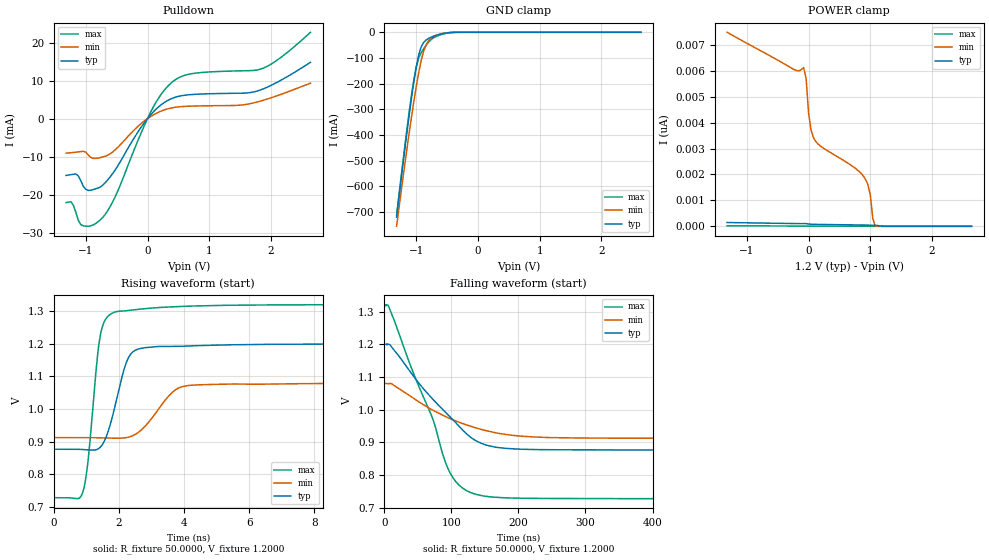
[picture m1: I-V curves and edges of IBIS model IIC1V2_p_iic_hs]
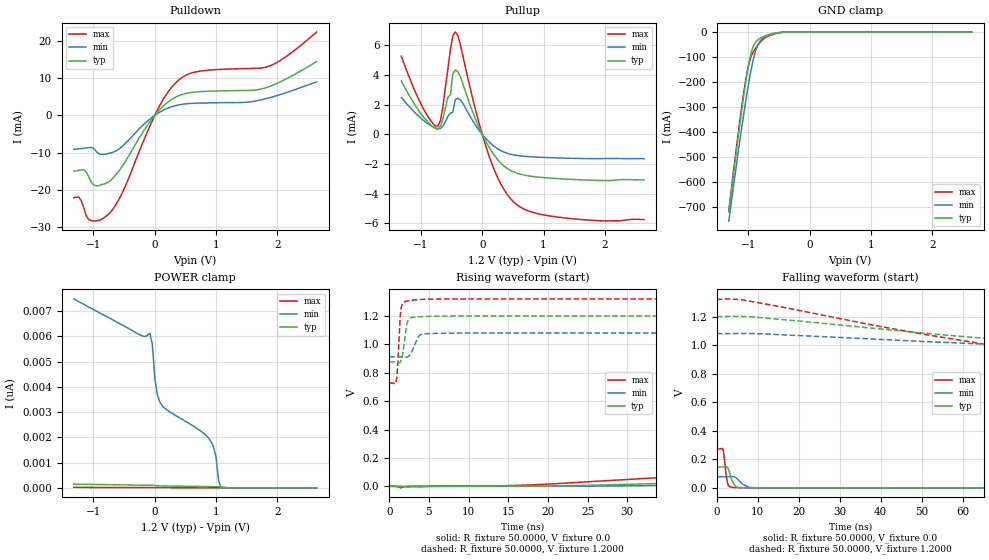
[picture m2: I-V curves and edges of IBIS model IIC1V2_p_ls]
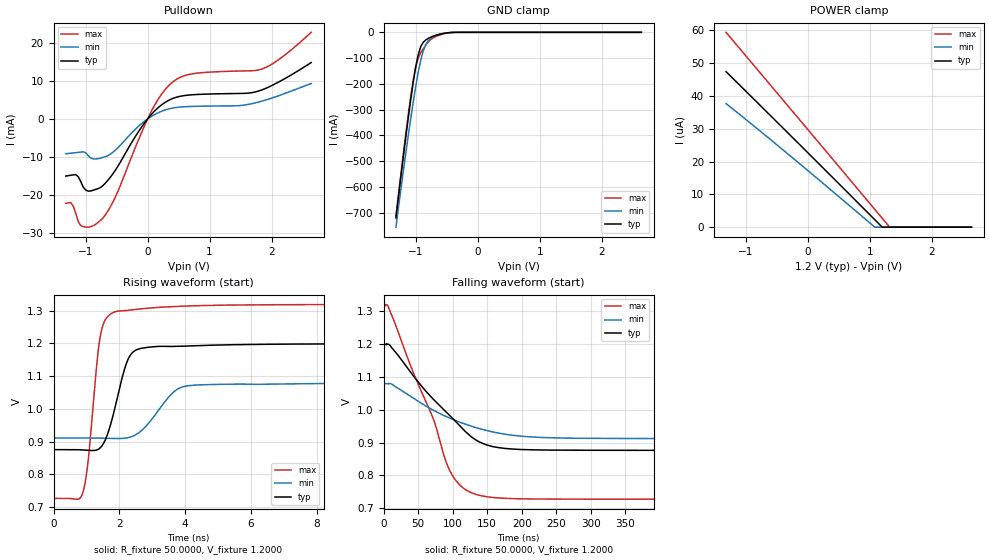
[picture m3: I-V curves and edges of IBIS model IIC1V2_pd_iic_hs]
| IBIS file qfn48_1p2v.ibs generated by Viper version: 2020.12.17
[IBIS Ver]   5.0
[Comment Char]   |_char
[File Name]   qfn48_1p2v.ibs
[File Rev]   1.3
[Date]   Thu Dec 17 17:48:23 2020
[Source]   NXP Viper 2020.12.17
[Notes]
[Disclaimer] IMPORTANT NOTICE
  This information is provided on an AS IS basis and without warranty.
  IN NO EVENT SHALL NXP BE LIABLE FOR INCIDENTAL OR CONSEQUENTIAL
  DAMAGES ARISING FROM USE OF THIS INFORMATION. THIS DISCLAIMER OF
  WARRANTY EXTENDS TO THE USER OF THE INFORMATION, AND TO THEIR CUSTOMERS
  OR USERS OF PRODUCTS  AND IS IN LIEU OF ALL WARRANTIES WHETHER EXPRESS,
  IMPLIED, OR STATUTORY, INCLUDING IMPLIED WARRANTIES OF MERCHANTABILITY
  OR FITNESS FOR PARTICULAR PURPOSE.
  NXP does not represent or warrant that the information furnished
  hereunder is free of infringement of any third party patents,
  copyrights, trade secrets, or other intellectual property rights.
  NXP does not represent or warrant that the information is free of
  defect, or that it meets any particular standard, requirements or need
  of the user of the infomation or their customers.
  NXP reserves the right to change the information in this file
  without notice.
   http://www.nxp.com
[Copyright]   (C) Copyright NXP 2004 - 2020, All Rights Reserved.
|   qfn48
[Component]   qfn48
[Manufacturer]   NXP
[Package]
| variable   typ   min   max
R_pkg   0.17546   0.085233   0.21913
L_pkg   1.979e-9   1.305e-9   2.456e-9
C_pkg   2.005e-13   1.705e-13   3.136e-13
[Pin] signal_name   model_name   R_pin   L_pin   C_pin
1   OPAMP2_INN   NC   0.19686   2.31e-9   1.975e-13
2   P0_1   gpio   0.19885   2.125e-9  1.995e-13
3   P1_0   gpio   0.18462   1.924e-9  1.916e-13
4   P0_11   gpio   0.16868   1.868e-9  1.705e-13
5   VDDIO_1   POWER   NA   NA   NA
6   VDDA   POWER   NA   NA   NA
7   VREF_OUT   NC   0.085233  1.305e-9  2.26e-13
8   VREFP   NC   0.088717  1.309e-9  2.417e-13
9   VREFN   GND   NA   NA   NA
10   P0_16   gpio   0.17435   1.987e-9  1.764e-13
11   P0_10   gpio   0.18496   2.194e-9  1.962e-13
12   P0_15   gpio   0.20527   2.456e-9  2.081e-13
13   P0_8   gpio   0.19119   2.293e-9  1.955e-13
14   OPAMP0_INN   NC   0.1741   2.073e-9  2.101e-13
15   P0_27   gpio   0.16311   1.909e-9  1.814e-13
16   OPAMP1_INN   NC   0.16129   1.801e-9  1.909e-13
17   RESETN   gpio   0.16527   1.717e-9  1.895e-13
18   VDD_CORE   POWER   NA   NA   NA
19   P0_17   gpio   0.16074   1.801e-9  1.861e-13
20   P0_7   gpio   0.1631   1.762e-9  1.925e-13
21   VDDIO_1   POWER   NA   NA   NA
22   VSS_MAIN   GND   NA   NA   NA
23   LX   NC   0.10755   1.361e-9  3.136e-13
24   VDD_MAIN_PWR   NC   NA   NA   NA
25   VBAT   NC   0.21039   2.199e-9  2.126e-13
26   P0_0   gpio   0.19752   2.015e-9  2.122e-13
27   P0_9   gpio   0.17432   1.951e-9  1.886e-13
28   P0_18   gpio   0.16396   1.852e-9  1.719e-13
29   P1_1   gpio   0.1654   1.786e-9  1.75e-13
30   P0_26   gpio   0.16144   1.856e-9  1.764e-13
31   P1_2   gpio   0.16991   1.948e-9  1.848e-13
32   P1_3   gpio   0.18887   2.054e-9  1.928e-13
33   P0_24   gpio   0.17001   1.885e-9  1.791e-13
34   P0_13   iic   0.18016   2.084e-9  1.944e-13
35   P0_14   iic   0.19867   2.298e-9  2.017e-13
36   P0_20   gpio   0.21913   2.324e-9  2.127e-13
37   P0_21   gpio   0.20869   2.216e-9  2.193e-13
38   P0_2   gpio   0.21473   2.265e-9  2.308e-13
39   P0_19   gpio   0.18997   2.14e-9   2.172e-13
40   P0_3   gpio   0.17488   1.926e-9  2.022e-13
41   VDDIO_2   POWER   NA   NA   NA
42   P0_4   gpio   0.16342   1.796e-9  1.814e-13
43   P0_6   gpio   0.16772   1.736e-9  1.992e-13
44   P0_5   gpio   0.16504   1.891e-9  1.879e-13
45   P0_29   gpio   0.16929   1.996e-9  1.98e-13
46   P1_11   gpio   0.18558   2.171e-9  1.964e-13
47   P0_30   gpio   0.20664   2.318e-9  2.205e-13
48   P2_1   gpio   0.1989   2.278e-9  1.972e-13
49   VSS   GND   NA   NA   NA
[Pin Mapping]   pulldown_ref   pullup_ref
1   NC   NC
2   VSS   VDDA
3   VSS   VDDA
4   VSS   VDDA
5   NC   VDDIO_1
6   NC   VDDA
7   NC   NC
8   NC   NC
9   VREFN   NC
10   VSS   VDDA
11   VSS   VDDA
12   VSS   VDDA
13   VSS   VDDA
14   NC   NC
15   VSS   VDDA
16   NC   NC
17   VSS   VDDIO_1
18   NC   VDD_CORE
19   VSS   VDDIO_1
20   VSS   VDDIO_1
21   NC   VDDIO_1
22   VSS_MAIN   NC
23   NC   NC
24   NC   NC
25   NC   NC
26   VSS   VDDIO_2
27   VSS   VDDIO_2
28   VSS   VDDIO_2
29   VSS   VDDIO_2
30   VSS   VDDIO_2
31   VSS   VDDIO_2
32   VSS   VDDIO_2
33   VSS   VDDIO_2
34   VSS   VDDIO_2
35   VSS   VDDIO_2
36   VSS   VDDIO_2
37   VSS   VDDIO_2
38   VSS   VDDIO_2
39   VSS   VDDIO_2
40   VSS   VDDIO_2
41   NC   VDDIO_2
42   VSS   VDDIO_2
43   VSS   VDDIO_2
44   VSS   VDDIO_2
45   VSS   VDDIO_2
46   VSS   VDDIO_2
47   VSS   VDDIO_2
48   VSS   VDDA
49   VSS   NC
|*   Model Selector   *
[Model Selector] gpio
MFIO1V2_pd_hs   EPUN=1 EPD=1 EHS=1
MFIO1V2_pd_ls   EPUN=1 EPD=1 EHS=0
MFIO1V2_pu_hs   EPUN=0 EPD=0 EHS=1
MFIO1V2_pu_ls   EPUN=0 EPD=0 EHS=0
MFIO1V2_p_hs   EPUN=1 EPD=0 EHS=1
MFIO1V2_p_ls   EPUN=1 EPD=0 EHS=0
MFIO1V2_r_hs   EPUN=0 EPD=1 EHS=1
MFIO1V2_r_ls   EPUN=0 EPD=1 EHS=0
[Model Selector] iic
IIC1V2_pd_hs   EGP=1 EPUN=1 EPD=1 EHS=1
IIC1V2_pd_ls   EGP=1 EPUN=1 EPD=1 EHS=0
IIC1V2_p_hs   EGP=1 EPUN=1 EPD=0 EHS=1
IIC1V2_p_ls   EGP=1 EPUN=1 EPD=0 EHS=0
IIC1V2_pu_hs   EGP=1 EPUN=0 EPD=0 EHS=1
IIC1V2_pu_ls   EGP=1 EPUN=0 EPD=0 EHS=0
IIC1V2_r_hs   EGP=1 EPUN=0 EPD=1 EHS=1
IIC1V2_r_ls   EGP=1 EPUN=0 EPD=1 EHS=0
IIC1V2_pd_iic_hs   EGP=0 ECS=0 EPUN=1 EPD=1
IIC1V2_p_iic_hs   EGP=0 ECS=0 EPUN=1 EPD=0
IIC1V2_pu_iic_hs   EGP=0 ECS=0 EPUN=0 EPD=0
IIC1V2_r_iic_hs   EGP=0 ECS=0 EPUN=0 EPD=1
IIC1V2_pd_iic_pu_hs   EGP=0 ECS=1 EPUN=1 EPD=1 SSEL=1
IIC1V2_p_iic_pu_hs   EGP=0 ECS=1 EPUN=1 EPD=0 SSEL=1
IIC1V2_pu_iic_pu_hs   EGP=0 ECS=1 EPUN=0 EPD=0 SSEL=1
IIC1V2_r_iic_pu_hs   EGP=0 ECS=1 EPUN=0 EPD=1 SSEL=1
| End [Component] qfn48
| Models and submodels in the file (24): IIC1V2_p_hs (I/O), IIC1V2_p_iic_hs (I/O_open_drain), IIC1V2_p_iic_pu_hs (I/O_open_drain), IIC1V2_p_ls (I/O), IIC1V2_pd_hs (I/O), IIC1V2_pd_iic_hs (I/O_open_drain), IIC1V2_pd_iic_pu_hs (I/O_open_drain), IIC1V2_pd_ls (I/O), IIC1V2_pu_hs (I/O), IIC1V2_pu_iic_hs (I/O_open_drain), IIC1V2_pu_iic_pu_hs (I/O_open_drain), IIC1V2_pu_ls (I/O), IIC1V2_r_hs (I/O), IIC1V2_r_iic_hs (I/O_open_drain), IIC1V2_r_iic_pu_hs (I/O_open_drain), IIC1V2_r_ls (I/O), MFIO1V2_p_hs (I/O), MFIO1V2_p_ls (I/O), MFIO1V2_pd_hs (I/O), MFIO1V2_pd_ls (I/O), MFIO1V2_pu_hs (I/O), MFIO1V2_pu_ls (I/O), MFIO1V2_r_hs (I/O), MFIO1V2_r_ls (I/O)
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[Model] IIC1V2_p_iic_hs
|   Model IIC1V2_p_iic_hs
| This model was characterised for following simulation conditions:
| External (pad) voltage:
|   - Typ: 1.2V,   - Min: 1.08V,   - Max: 1.32V
| Library cells for typ/min/max conditions are connected as defined below:
|  IO - External Pad
|  A - Core Input
|  EN - Output Buffer Enable
|  BOOST - vdde
|  ECS - gnd
|  EGP - gnd
|  ENZI - vdd
|  EPD - gnd
|  EPUN - vdd
|  ZI - NC
|  ZIF - NC
|  gnd - gnd
|  gnde - gnde
|  vdd - vdd
|  vdde - vdde
| All other pins connected to ground
Model_type I/O_open_drain
Polarity   Non-Inverting
Enable   Active-Low
Vinl =   0.5400V
Vinh =   1.2600V
Vmeas =  0.9000V
Cref =   0.0F
Rref =   1.0000k
Vref =   1.2000V
C_comp   3.6477pF   3.5140pF   3.7674pF
|C_comp_pullup   0.9543pF   0.9094pF   0.9729pF
|C_comp_pulldown   2.3399pF   2.4911pF   2.1962pF
[Model Spec]
| variable   typ   min   max
Vinh   0.3600V   0.3240V   0.3960V
Vinl   0.8400V   0.7560V   0.9240V
Vmeas   0.6000V   0.5400V   0.6600V
Vref   1.2000V   1.0800V   1.3200V
Cref   0.0F   0.0F   0.0F
Rref   1.0000k   1.0000k   1.0000k
[Temperature Range]   25.0000   0.1250k   -40.0000
[Voltage Range]   1.2000V   1.0800V   1.3200V
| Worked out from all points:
|   slope of the pulldown table from 0 to 0.18 V, typ, clamps not added: 58.3 ohm
|   GND clamp passes 1 mA (typ) near -0.45 V on its own axis
|   rising waveform, R_fixture 50.0000, V_fixture 1.2000: 20-80 % time 502ps typ, 802ps min, 333ps max; typ from 0.877 V to 1.2 V
|   falling waveform, R_fixture 50.0000, V_fixture 1.2000: 20-80 % time 83.3ns typ, 98.9ns min, 62.7ns max; typ from 1.2 V to 0.877 V
[Pulldown]
|Voltage   I(typ)   I(min)   I(max)
-1.32V    -14.96mA   -9.099mA   -22.09mA
-1.24V    -14.75mA   -8.982mA   -21.89mA
-1.16V    -14.56mA   -8.83mA    -24.7mA
-1.04V    -17.82mA   -8.609mA   -28.21mA
-920mV    -18.88mA   -10.21mA   -28.21mA
-720mV    -17.44mA   -10.07mA   -25.94mA
-520mV    -13.41mA   -8.157mA   -20.44mA
80mV      1.521mA    840uA      2.628mA
440mV     5.569mA    2.951mA    10.1mA
760mV     6.377mA    3.307mA    11.92mA
1.84V     7.596mA    4.654mA    13.07mA
2.64V     14.81mA    9.301mA    22.71mA
[GND_clamp]
|Voltage   I(typ)   I(min)   I(max)
-1.32V    -720.7mA   -756.4mA   -713.8mA
-1.12V    -330.9mA   -399.5mA   -316.8mA
-1.04V    -192.4mA   -269.2mA   -184.4mA
-1V       -133.6mA   -209.3mA   -133.5mA
-960mV    -86.73mA   -154.7mA   -99.45mA
-920mV    -55.68mA   -108.2mA   -79.01mA
-880mV    -39.01mA   -72.34mA   -63.7mA
-840mV    -29.9mA    -47.99mA   -50.25mA
-760mV    -18.92mA   -23.38mA   -28.31mA
-640mV    -9.212mA   -8.622mA   -12.72mA
-400mV    -328.4uA   -396.6uA   -434.3uA
2.64V     0A         0A         0A
[POWER_clamp]
|Voltage   I(typ)   I(min)   I(max)
-1.32V    146.2pA    7.487nA    20.6pA
-240mV    107.2pA    6.058nA    10.71pA
-80mV     104.3pA    6.128nA    10.43pA
-40mV     105.3pA    5.7nA      9.002pA
0V        87.49pA    4.363nA    8.131pA
80mV      77.4pA     3.412nA    7.54pA
880mV     48.09pA    1.964nA    2.626pA
960mV     44.51pA    1.611nA    2.139pA
1V        42.37pA    1.211nA    1.894pA
1.04V     39.75pA    304.3pA    1.646pA
1.08V     36.09pA    0A         1.394pA
2.64V     0A         0A         0A
[Ramp]
| variable   typ   min   max
dV/dt_r  0.1940/0.5018n   0.1007/0.8020n   0.3553/0.3326n
dV/dt_f  0.1940/83.3256n   0.1006/98.9726n   0.3552/62.6671n
R_load = 50.0000
[Rising Waveform]
R_fixture= 50.0000
V_fixture= 1.2000
V_fixture_min= 1.0800
V_fixture_max= 1.3200
|time   V(typ)   V(min)   V(max)
0s        876.6mV    912.2mV    727.9mV
906ps     875.6mV    912.3mV    750.4mV
1.06ns    874.5mV    912.2mV    848.8mV
1.379ns   878.7mV    911.7mV    1.194V
1.659ns   928.2mV    911mV      1.284V
2.166ns   1.124V     911.3mV    1.301V
2.479ns   1.179V     920.8mV    1.304V
3.849ns   1.192V     1.065V     1.314V
6.228ns   1.198V     1.076V     1.319V
1us       1.2V       1.08V      1.32V
[Falling Waveform]
R_fixture= 50.0000
V_fixture= 1.2000
V_fixture_min= 1.0800
V_fixture_max= 1.3200
|time   V(typ)   V(min)   V(max)
0s        1.2V       1.08V      1.32V
6.631ns   1.2V       1.079V     1.315V
39.25ns   1.114V     1.041V     1.133V
72.68ns   1.031V     998mV      969.3mV
95.48ns   983.6mV    975mV      817.5mV
111.3ns   949.7mV    961.8mV    769.6mV
133.6ns   908.9mV    946.1mV    743.1mV
169.3ns   884.4mV    928.2mV    731.8mV
230ns     878mV      916mV      728.8mV
1us       876.7mV    912.3mV    728mV
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[Model] IIC1V2_p_ls
|   Model IIC1V2_p_ls
| This model was characterised for following simulation conditions:
| External (pad) voltage:
|   - Typ: 1.2V,   - Min: 1.08V,   - Max: 1.32V
| Library cells for typ/min/max conditions are connected as defined below:
|  IO - External Pad
|  A - Core Input
|  EN - Output Buffer Enable
|  BOOST - vdde
|  EGP - vdd
|  EHS - gnd
|  ENZI - vdd
|  EPD - gnd
|  EPUN - vdd
|  ZI - NC
|  ZIF - NC
|  gnd - gnd
|  gnde - gnde
|  vdd - vdd
|  vdde - vdde
| All other pins connected to ground
Model_type I/O
Polarity   Non-Inverting
Enable   Active-Low
Vinl =   0.5400V
Vinh =   1.2600V
Vmeas =  0.9000V
Cref =   0.0F
Rref =   1.0000k
Vref =   0.0V
C_comp   3.6473pF   3.5138pF   3.7665pF
|C_comp_pullup   0.9537pF   0.9078pF   0.9727pF
|C_comp_pulldown   2.3401pF   2.4920pF   2.1963pF
[Model Spec]
| variable   typ   min   max
Vinh   0.3600V   0.3240V   0.3960V
Vinl   0.8400V   0.7560V   0.9240V
Vmeas   0.6000V   0.5400V   0.6600V
[Temperature Range]   25.0000   0.1250k   -40.0000
[Voltage Range]   1.2000V   1.0800V   1.3200V
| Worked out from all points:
|   slope of the pulldown table from 0 to 0.18 V, typ, clamps not added: 58.3 ohm
|   slope of the pullup table from 0 to 0.18 V, typ, clamps not added: 138 ohm
|   GND clamp passes 1 mA (typ) near -0.45 V on its own axis
|   rising waveform, R_fixture 50.0000, V_fixture 0.0: 20-80 % time 73.3ns typ, 82.8ns min, 61.7ns max; typ from 0 V to 0.146 V
|   rising waveform, R_fixture 50.0000, V_fixture 1.2000: 20-80 % time 495ps typ, 787ps min, 328ps max; typ from 0.877 V to 1.2 V
|   falling waveform, R_fixture 50.0000, V_fixture 0.0: 20-80 % time 1.12ns typ, 1.9ns min, 700ps max; typ from 0.146 V to 0 V
|   falling waveform, R_fixture 50.0000, V_fixture 1.2000: 20-80 % time 83.3ns typ, 98.9ns min, 62.7ns max; typ from 1.2 V to 0.877 V
[Pulldown]
|Voltage   I(typ)   I(min)   I(max)
-1.32V    -14.96mA   -9.099mA   -22.09mA
-1.24V    -14.75mA   -8.982mA   -21.89mA
-1.16V    -14.56mA   -8.83mA    -24.7mA
-1.04V    -17.82mA   -8.609mA   -28.21mA
-920mV    -18.88mA   -10.21mA   -28.21mA
-720mV    -17.44mA   -10.07mA   -25.94mA
-520mV    -13.41mA   -8.157mA   -20.44mA
80mV      1.521mA    840uA      2.628mA
440mV     5.569mA    2.951mA    10.1mA
760mV     6.377mA    3.307mA    11.92mA
1.84V     7.559mA    4.586mA    13.06mA
2.64V     14.43mA    8.958mA    22.36mA
[Pullup]
|Voltage   I(typ)   I(min)   I(max)
-1.32V    3.599mA    2.494mA    5.272mA
-960mV    1.183mA    954.7uA    1.735mA
-720mV    366.8uA    380.1uA    560.7uA
-640mV    1.076mA    572uA      1.919mA
-520mV    2.672mA    1.434mA    5.709mA
-480mV    4.096mA    1.502mA    6.65mA
-440mV    4.343mA    2.346mA    6.902mA
120mV     -924.8uA   -536.9uA   -1.554mA
360mV     -2.143mA   -1.197mA   -3.751mA
600mV     -2.653mA   -1.434mA   -4.838mA
1.36V     -3.007mA   -1.596mA   -5.631mA
2.64V     -3.069mA   -1.636mA   -5.736mA
[GND_clamp]
|Voltage   I(typ)   I(min)   I(max)
-1.32V    -720.7mA   -756.4mA   -713.8mA
-1.12V    -330.9mA   -399.5mA   -316.8mA
-1.04V    -192.4mA   -269.2mA   -184.4mA
-1V       -133.6mA   -209.3mA   -133.5mA
-960mV    -86.73mA   -154.7mA   -99.45mA
-920mV    -55.68mA   -108.2mA   -79.01mA
-880mV    -39.01mA   -72.34mA   -63.7mA
-840mV    -29.9mA    -47.99mA   -50.25mA
-760mV    -18.92mA   -23.38mA   -28.31mA
-640mV    -9.212mA   -8.622mA   -12.72mA
-400mV    -328.4uA   -396.6uA   -434.3uA
2.64V     0A         0A         0A
[POWER_clamp]
|Voltage   I(typ)   I(min)   I(max)
-1.32V    146.2pA    7.487nA    20.6pA
-240mV    107.2pA    6.058nA    10.71pA
-80mV     104.3pA    6.128nA    10.43pA
-40mV     105.3pA    5.7nA      9.002pA
0V        87.49pA    4.363nA    8.131pA
80mV      77.4pA     3.412nA    7.54pA
880mV     48.09pA    1.964nA    2.626pA
960mV     44.51pA    1.611nA    2.139pA
1V        42.37pA    1.211nA    1.894pA
1.04V     39.75pA    304.3pA    1.646pA
1.08V     36.09pA    0A         1.394pA
2.64V     0A         0A         0A
[Ramp]
| variable   typ   min   max
dV/dt_r  87.7367m/73.3638n   46.3941m/82.7765n   0.1636/61.7560n
dV/dt_f  0.1940/83.2849n   0.1006/98.9600n   0.3552/62.6860n
R_load = 50.0000
[Rising Waveform]
R_fixture= 50.0000
V_fixture= 0.0
V_fixture_min= 0.0
V_fixture_max= 0.0
|time   V(typ)   V(min)   V(max)
0s        663.7pV    60.46nV    39.17pV
1.445ns   -661.9uV   126.7uV    -10.83mV
2.434ns   -6.509mV   -500.2uV   -616.3uV
18.13ns   1.187mV    309.2uV    10.36mV
57.57ns   55.19mV    22.26mV    135.2mV
97.04ns   102.6mV    47.31mV    224.2mV
116.5ns   119mV      56.56mV    249.1mV
149ns     135.6mV    67.15mV    265.8mV
252.5ns   145.7mV    76.41mV    272.5mV
1us       146.2mV    77.32mV    272.7mV
[Rising Waveform]
R_fixture= 50.0000
V_fixture= 1.2000
V_fixture_min= 1.0800
V_fixture_max= 1.3200
|time   V(typ)   V(min)   V(max)
0s        876.6mV    912.2mV    727.9mV
902.2ps   874.8mV    912.4mV    743.3mV
1.062ns   872.6mV    912.3mV    843.4mV
1.394ns   875.4mV    911.3mV    1.202V
1.67ns    926.1mV    909.9mV    1.286V
2.162ns   1.12V      908.9mV    1.304V
2.466ns   1.178V     917.1mV    1.308V
3.862ns   1.194V     1.065V     1.315V
6.134ns   1.198V     1.077V     1.319V
1us       1.2V       1.08V      1.32V
[Falling Waveform]
R_fixture= 50.0000
V_fixture= 0.0
V_fixture_min= 0.0
V_fixture_max= 0.0
|time   V(typ)   V(min)   V(max)
0s        146.3mV    77.36mV    272.8mV
1.538ns   146.4mV    77.36mV    268.8mV
1.722ns   147mV      77.34mV    240.2mV
2.304ns   148.8mV    77.28mV    90.92mV
2.892ns   127.1mV    77.84mV    15.63mV
4.35ns    19.3mV     76.26mV    1.996mV
5.878ns   1.798mV    37.55mV    745.5uV
7.946ns   487.2uV    4.089mV    481.2uV
12.72ns   263uV      265.1uV    241.1uV
1us       25.89nV    103.3nV    14.92nV
[Falling Waveform]
R_fixture= 50.0000
V_fixture= 1.2000
V_fixture_min= 1.0800
V_fixture_max= 1.3200
|time   V(typ)   V(min)   V(max)
0s        1.2V       1.08V      1.32V
6.433ns   1.2V       1.081V     1.316V
43.29ns   1.103V     1.035V     1.112V
71.43ns   1.034V     999.5mV    976.4mV
96ns      982.7mV    974.6mV    815.2mV
113.7ns   944.6mV    960.1mV    765.2mV
137ns     904.7mV    944.2mV    741.1mV
175.9ns   882.8mV    926mV      731mV
266.1ns   877.4mV    914mV      728.5mV
1us       876.7mV    912.3mV    728mV
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[Model] IIC1V2_pd_iic_hs
|   Model IIC1V2_pd_iic_hs
| This model was characterised for following simulation conditions:
| External (pad) voltage:
|   - Typ: 1.2V,   - Min: 1.08V,   - Max: 1.32V
| Library cells for typ/min/max conditions are connected as defined below:
|  IO - External Pad
|  A - Core Input
|  EN - Output Buffer Enable
|  BOOST - vdde
|  ECS - gnd
|  EGP - gnd
|  ENZI - vdd
|  EPD - vdd
|  EPUN - vdd
|  ZI - NC
|  ZIF - NC
|  gnd - gnd
|  gnde - gnde
|  vdd - vdd
|  vdde - vdde
| All other pins connected to ground
Model_type I/O_open_drain
Polarity   Non-Inverting
Enable   Active-Low
Vinl =   0.5400V
Vinh =   1.2600V
Vmeas =  0.9000V
Cref =   0.0F
Rref =   1.0000k
Vref =   1.2000V
C_comp   3.6168pF   3.4770pF   3.7425pF
|C_comp_pullup   0.9409pF   0.9008pF   0.9551pF
|C_comp_pulldown   2.3238pF   2.4763pF   2.1787pF
[Model Spec]
| variable   typ   min   max
Vinh   0.3600V   0.3240V   0.3960V
Vinl   0.8400V   0.7560V   0.9240V
Vmeas   0.6000V   0.5400V   0.6600V
Vref   1.2000V   1.0800V   1.3200V
Cref   0.0F   0.0F   0.0F
Rref   1.0000k   1.0000k   1.0000k
[Temperature Range]   25.0000   0.1250k   -40.0000
[Voltage Range]   1.2000V   1.0800V   1.3200V
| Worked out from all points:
|   slope of the pulldown table from 0 to 0.18 V, typ, clamps not added: 58.3 ohm
|   GND clamp passes 1 mA (typ) near -0.45 V on its own axis
|   rising waveform, R_fixture 50.0000, V_fixture 1.2000: 20-80 % time 501ps typ, 801ps min, 332ps max; typ from 0.876 V to 1.2 V
|   falling waveform, R_fixture 50.0000, V_fixture 1.2000: 20-80 % time 83.2ns typ, 98.9ns min, 62.5ns max; typ from 1.2 V to 0.876 V
[Pulldown]
|Voltage   I(typ)   I(min)   I(max)
-1.32V    -14.96mA   -9.099mA   -22.09mA
-1.24V    -14.75mA   -8.982mA   -21.89mA
-1.16V    -14.56mA   -8.83mA    -24.7mA
-1.04V    -17.82mA   -8.609mA   -28.21mA
-920mV    -18.88mA   -10.21mA   -28.21mA
-720mV    -17.44mA   -10.07mA   -25.94mA
-520mV    -13.41mA   -8.157mA   -20.44mA
80mV      1.521mA    840uA      2.628mA
440mV     5.569mA    2.951mA    10.1mA
760mV     6.377mA    3.307mA    11.92mA
1.84V     7.592mA    4.649mA    13.07mA
2.64V     14.79mA    9.287mA    22.7mA
[GND_clamp]
|Voltage   I(typ)   I(min)   I(max)
-1.32V    -720.7mA   -756.5mA   -713.8mA
-1.12V    -330.9mA   -399.5mA   -316.8mA
-1.04V    -192.4mA   -269.2mA   -184.4mA
-1V       -133.6mA   -209.3mA   -133.5mA
-960mV    -86.74mA   -154.7mA   -99.46mA
-920mV    -55.69mA   -108.2mA   -79.02mA
-880mV    -39.02mA   -72.35mA   -63.71mA
-840mV    -29.9mA    -48mA      -50.26mA
-760mV    -18.93mA   -23.39mA   -28.32mA
-640mV    -9.22mA    -8.628mA   -12.73mA
-400mV    -335.3uA   -402.3uA   -442.6uA
2.64V     0A         0A         0A
[POWER_clamp]
|Voltage   I(typ)   I(min)   I(max)
-1.32V    47.4uA     37.67uA    59.39uA
-280mV    27.94uA    21.65uA    36.04uA
1.08V     2.274uA    0A         5.413uA
1.2V      0A         0A         2.707uA
1.32V     0A         0A         0A
2.64V     0A         0A         0A
[Ramp]
| variable   typ   min   max
dV/dt_r  0.1938/0.5014n   0.1006/0.8017n   0.3548/0.3320n
dV/dt_f  0.1938/83.2106n   0.1006/98.8181n   0.3548/62.5201n
R_load = 50.0000
[Rising Waveform]
R_fixture= 50.0000
V_fixture= 1.2000
V_fixture_min= 1.0800
V_fixture_max= 1.3200
|time   V(typ)   V(min)   V(max)
0s        875.8mV    911.4mV    727.2mV
907ps     874.8mV    911.6mV    750.1mV
1.062ns   873.7mV    911.5mV    850mV
1.381ns   878mV      911mV      1.195V
1.661ns   928.2mV    910.2mV    1.284V
2.17ns    1.125V     910.6mV    1.3V
2.483ns   1.178V     920.3mV    1.303V
3.857ns   1.191V     1.065V     1.313V
6.11ns    1.197V     1.075V     1.317V
1us       1.199V     1.079V     1.319V
[Falling Waveform]
R_fixture= 50.0000
V_fixture= 1.2000
V_fixture_min= 1.0800
V_fixture_max= 1.3200
|time   V(typ)   V(min)   V(max)
0s        1.199V     1.079V     1.319V
6.361ns   1.199V     1.079V     1.315V
41.12ns   1.108V     1.037V     1.122V
69.41ns   1.037V     1.001V     985.5mV
95.48ns   982.5mV    974.3mV    816mV
113.6ns   943.7mV    959.3mV    764.4mV
136.9ns   903.6mV    943.3mV    740.3mV
174.6ns   882.2mV    925.6mV    730.4mV
268.4ns   876.6mV    913.2mV    727.7mV
1us       875.9mV    911.5mV    727.2mV
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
